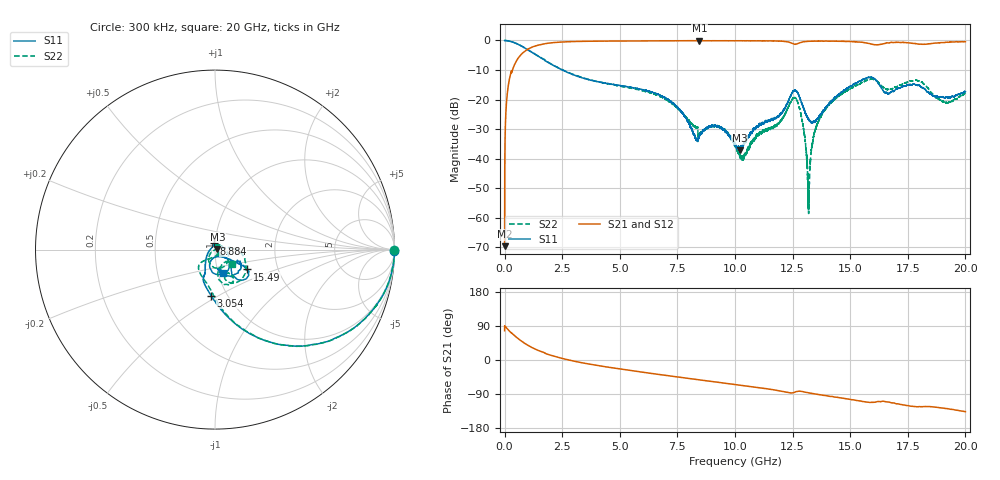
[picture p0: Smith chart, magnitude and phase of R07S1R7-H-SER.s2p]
!{R07S1R7}
!Johanson Technology Inc.
!www.johansontechnology.com
!Test Board Conditions:
!Substrate Type  RO4350B
!Substrate Thickness  10 mil
!Substrate Dk  3.66
!TL Type: GCPW
!TL Trace Width  21 mil
!TL Gap  20 mil
!Electrode orientation  Horizontal
!DUT TOPOLOGY	SERIES
!Mounting Pad LxW  16x21 mil
! Created Sat Feb  6 11:22:06 2021
# hz S ma R 50
! 2 Port Network Data from SP1.SP block
! freq  magS11  angS11  magS21  angS21  magS12  angS12  magS22  angS22
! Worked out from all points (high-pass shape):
!   20001 points, 300 kHz to 20 GHz, reference 50 ohm
!   highest |S21| = -0.08 dB at 8.456 GHz (marker M1); lowest = -69.7 dB at 300 kHz (marker M2)
!   |S21| within 3 dB of the highest: 982.8 MHz to end of sweep
!   lowest |S11| = -37.2 dB at 10.21 GHz (marker M3), VSWR 1.03, Z = 51.3 + j0.386 ohm
!   |S11| at or under -10 dB: 2.504 GHz to end of sweep
!   |S22| runs from -58.6 to 0.0 dB; largest |S21 - S12| = 0.011
!   S11 on the Smith chart (normalised r, x): 300 kHz: open; 3.054 GHz: 0.84, -0.46; 8.884 GHz: 0.98, +0.07; 15.49 GHz: 1.40, -0.32; 20 GHz: 1.05, -0.28
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300000  0.9976 -0.4  0.0003287 77.2  0.0002934 87.5  0.9971 -0.3
1.013e8  0.9927 -6.8  0.1092 83.3  0.1094 83.4  0.9924 -6.8
1.283e8  0.9893 -8.6  0.1379 81.5  0.1378 81.7  0.9901 -8.7
4.643e8  0.9044 -26.9  0.414 62.6  0.4134 62.6  0.9062 -26.8
1.5333e9  0.5197 -66.4  0.8455 23.6  0.8473 23.4  0.5252 -65.6
3.0543e9  0.2568 -95.1  0.9588 -3.6  0.9597 -3.5  0.2588 -91.1
3.3343e9  0.2351 -98.9  0.9651 -6.9  0.9651 -7.0  0.2379 -94.2
6.6673e9  0.1218 -116.9  0.9842 -37.9  0.9845 -37.9  0.1164 -136.8
8.4563e9  0.02411 113.2  0.9913 -52.4  0.9894 -52.4  0.02595 -67.2
8.8843e9  0.03525 102.2  0.9896 -55.8  0.989 -55.8  0.03455 -55.2
1.00003e10  0.01821 48.9  0.9877 -64.6  0.989 -64.7  0.01626 -31.5
1.02133e10  0.01382 15.8  0.9878 -66.4  0.9871 -66.4  0.01125 -6.1
1.25723e10  0.1422 -68.6  0.8669 -85.4  0.8685 -85.5  0.108 -67.8
1.29053e10  0.08395 -110.4  0.9358 -83.0  0.9368 -83.1  0.04597 -133.0
1.31713e10  0.04763 -99.9  0.9662 -86.4  0.9664 -86.3  0.002846 -117.7
1.33343e10  0.03962 -81.1  0.9713 -88.1  0.9723 -88.2  0.01526 14.8
1.39053e10  0.07 -40.6  0.9766 -93.7  0.9746 -93.7  0.06668 10.5
1.54863e10  0.2112 -31.6  0.9364 -108.7  0.9321 -108.7  0.1937 -24.6
1.66673e10  0.1254 -34.7  0.9063 -110.8  0.9101 -111.3  0.1495 -63.8
1.78523e10  0.1757 -51.0  0.8827 -123.3  0.8847 -123.2  0.213 -68.6
1.91383e10  0.1082 -80.6  0.9296 -128.0  0.931 -127.7  0.08864 -59.2
2e10  0.1359 -71.3  0.9538 -136.2  0.9491 -136.3  0.1252 -41.1
